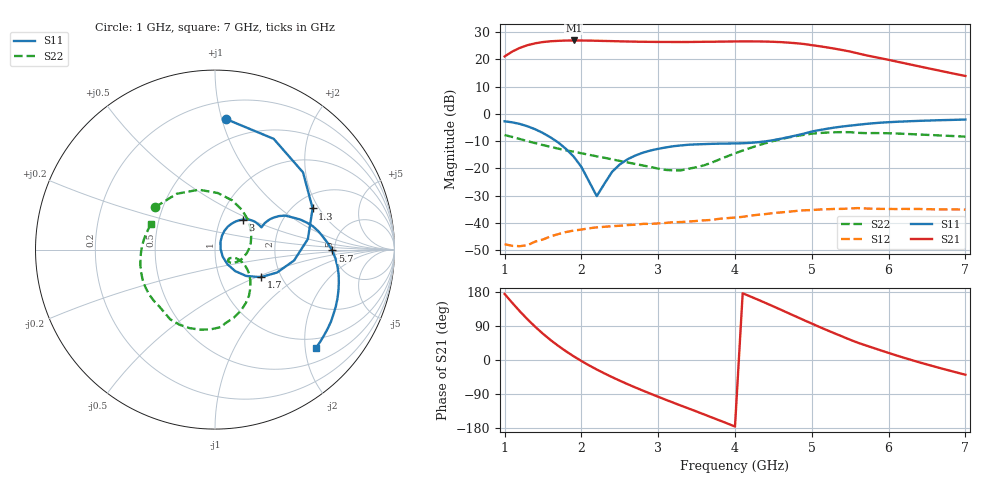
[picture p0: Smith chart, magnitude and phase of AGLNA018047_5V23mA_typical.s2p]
! Keysight Technologies,N5245B,MY58421923,A.15.40.11
! pna-50_lab Wed Jul 27 15:07:48 2022
# HZ S DB R 50
!freq (Hz)  S11DB  S11A  S21DB  S21A  S12DB  S12A  S22DB  S22A
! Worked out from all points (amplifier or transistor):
!   61 points, 1 GHz to 7 GHz, reference 50 ohm
!   highest |S21| = 26.9 dB at 1.9 GHz (marker M1)
!   |S21| within 3 dB of that: 1.178 GHz to 5.297 GHz (4.119 GHz wide, 127 % of centre)
!   unconditionally stable (mu >= 1): start of sweep to end of sweep
!   at 2 GHz: K = 2.93, MAG = 27.1 dB, |S12| = -42.4 dB
!   at 4 GHz: K = 1.85, MAG = 26.9 dB, |S12| = -38.0 dB
!   at 7 GHz: K = 2.03, MAG = 18.7 dB, |S12| = -35.1 dB
!   lowest NFmin = 0.60 dB at 3.3 GHz
!   S11 on the Smith chart (normalised r, x): 1 GHz: 0.33, +1.03; 1.3 GHz: 2.50, +1.76; 1.7 GHz: 1.58, -0.53; 3 GHz: 1.28, +0.45; 5.7 GHz: 4.76, -0.07; 7 GHz: 0.77, -2.22
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1e9  -2.73 85.3  21.01 174.3  -47.73 62.2  -7.77 144.8
1.1e9  -3.12 62.1  22.80 150.7  -48.33 61.8  -8.47 124.5
1.2e9  -3.71 41.3  24.16 128.1  -48.44 63.0  -9.23 105.2
1.3e9  -4.58 22.9  25.14 107.0  -48.05 67.4  -10.01 87.2
1.5e9  -7.03 -7.8  26.28 69.2  -45.97 66.6  -11.44 56.2
1.7e9  -10.52 -31.1  26.72 37.1  -44.01 60.1  -12.75 30.6
1.9e9  -15.68 -46.8  26.86 9.7  -42.73 52.2  -13.88 10.1
2e9  -19.42 -49.7  26.84 -2.6  -42.36 47.0  -14.44 1.4
2.3e9  -25.57 54.5  26.67 -35.4  -41.34 37.3  -16.08 -20.0
2.5e9  -18.52 63.3  26.54 -54.6  -40.96 30.6  -17.24 -30.4
2.7e9  -15.28 57.3  26.42 -72.3  -40.59 25.6  -18.35 -37.8
3e9  -12.80 46.9  26.32 -97.1  -40.10 17.9  -20.05 -41.2
3.5e9  -11.17 31.9  26.34 -136.0  -39.19 7.9  -19.53 -26.3
4e9  -10.83 25.6  26.50 -175.6  -37.97 -0.4  -14.48 -27.8
4.3e9  -10.39 27.1  26.50 159.1  -36.95 -7.6  -11.56 -41.7
4.6e9  -9.09 28.9  26.24 132.4  -36.08 -16.7  -9.27 -60.2
5e9  -6.48 22.0  25.13 96.1  -35.23 -30.8  -7.26 -86.0
5.4e9  -4.63 9.8  23.34 61.7  -34.79 -45.9  -6.69 -115.3
5.7e9  -3.70 -0.4  21.47 38.7  -34.64 -58.2  -7.06 -134.4
6e9  -3.06 -11.4  19.76 18.7  -34.81 -66.7  -7.12 -151.7
6.4e9  -2.57 -25.2  17.36 -6.2  -34.82 -78.4  -7.58 -173.5
7e9  -2.09 -44.4  13.86 -38.8  -35.06 -94.9  -8.35 158.1
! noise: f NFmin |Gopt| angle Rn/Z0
1e+09  2.434  0.3665  -46.34  0.5121
1.6e+09  1.137  0  90  0.0748
2.3e+09  0.8737  0  90  0.05571
3e+09  0.7128  0  90  0.04459
3.6e+09  0.825  0  90  0.0523
4.2e+09  0.7614  0.3175  7.603  0.1463
4.8e+09  1.101  0  90  0.07214
5.6e+09  1.18  0.2391  -25.7  0.5389
6.4e+09  1.401  0.4494  28.22  0.6402
7e+09  1.388  0.6528  48.4  0.7046
